(* Logix 5000 AddOnInstructionDefinition export AMP_Alarm_Code; software revision 20.04 *)

ADD_ON_INSTRUCTION AMP_Alarm_Code   (* revision 1.0 *)
// Applied Motion - Alarm Code - AOI
// Help:
// The Alarm Code AOI uses the raw data stored in the Alarm Code word (Element 1 from Input Assembly 0x65) to set individual appropriately named boolean outputs.
VAR_INPUT
   Input : DINT; {required}   // Element 1 from Drive Input Assembly (0x65)
END_VAR
VAR_OUTPUT
   Position_Limit : BOOL; {access Read Only, visible}
   CCW_Limit : BOOL; {access Read Only, visible}
   CW_Limit : BOOL; {access Read Only, visible}
   Over_Temp : BOOL; {access Read Only, visible}
   Excess_Regen_or_Internal_Voltage : BOOL; {access Read Only, visible}
   Over_Voltage : BOOL; {access Read Only, visible}
   Under_Voltage : BOOL; {access Read Only, visible}
   Over_Current : BOOL; {access Read Only, visible}
   Open_Motor_Windings : BOOL; {access Read Only, visible}
   Bad_Encoder : BOOL; {access Read Only, visible}
   Comm_Error : BOOL; {access Read Only, visible}
   Bad_Flash : BOOL; {access Read Only, visible}
   No_Move : BOOL; {access Read Only, visible}
   NA_1 : BOOL; {access Read Only, visible}
   Blank_Q_Segment : BOOL; {access Read Only, visible}
   NA_2 : BOOL; {access Read Only, visible}
END_VAR

ROUTINE Logic   (* ladder *)
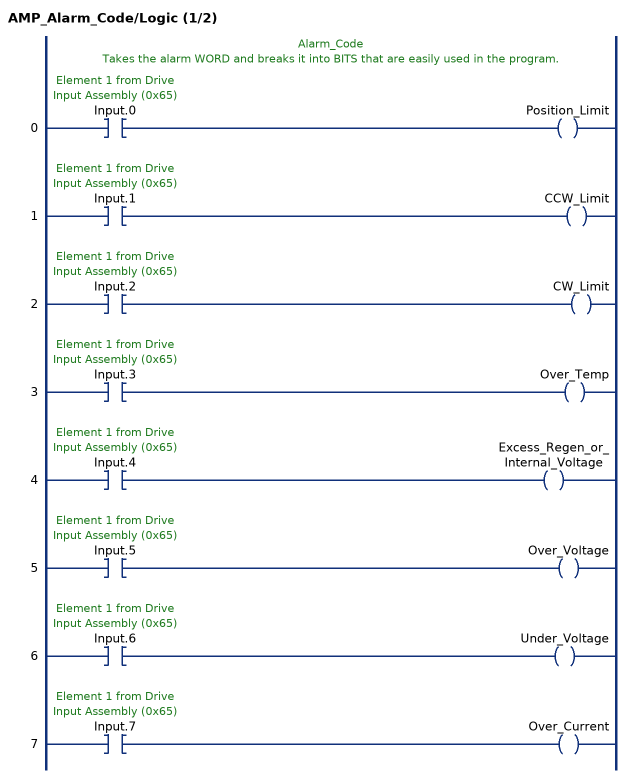
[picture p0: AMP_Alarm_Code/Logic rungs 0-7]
   // Alarm_Code
   // Takes the alarm WORD and breaks it into BITS that are easily used in the program.
   0: XIC(Input.0)OTE(Position_Limit);
   1: XIC(Input.1)OTE(CCW_Limit);
   2: XIC(Input.2)OTE(CW_Limit);
   3: XIC(Input.3)OTE(Over_Temp);
   4: XIC(Input.4)OTE(Excess_Regen_or_Internal_Voltage);
   5: XIC(Input.5)OTE(Over_Voltage);
   6: XIC(Input.6)OTE(Under_Voltage);
   7: XIC(Input.7)OTE(Over_Current);
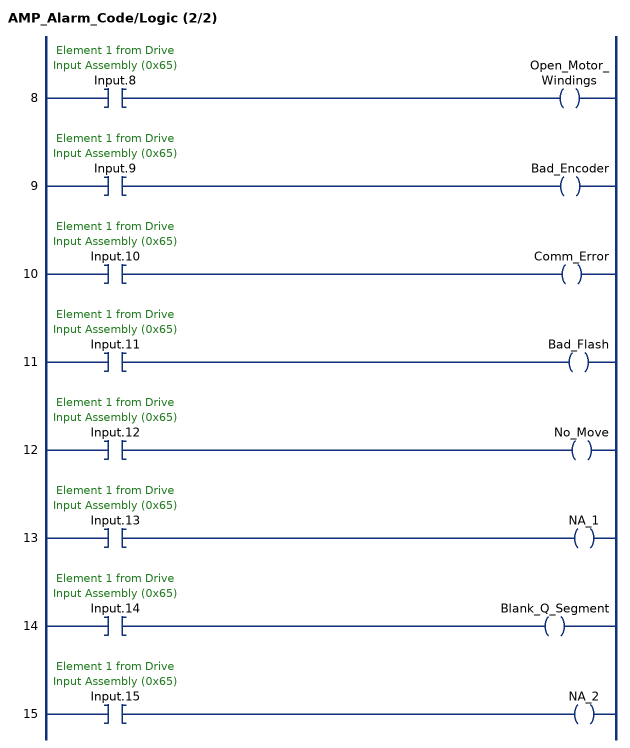
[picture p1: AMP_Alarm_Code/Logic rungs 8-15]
   8: XIC(Input.8)OTE(Open_Motor_Windings);
   9: XIC(Input.9)OTE(Bad_Encoder);
   10: XIC(Input.10)OTE(Comm_Error);
   11: XIC(Input.11)OTE(Bad_Flash);
   12: XIC(Input.12)OTE(No_Move);
   13: XIC(Input.13)OTE(NA_1);
   14: XIC(Input.14)OTE(Blank_Q_Segment);
   15: XIC(Input.15)OTE(NA_2);
END_ROUTINE
END_ADD_ON_INSTRUCTION
